PROGRAM p07_memoryCell
VAR
	S0: BOOL;
	S1: BOOL;
	L0: BOOL;
	L1: BOOL;
	L2: BOOL;
	RS_cell: RS;
	SR_cell: SR;
END_VAR

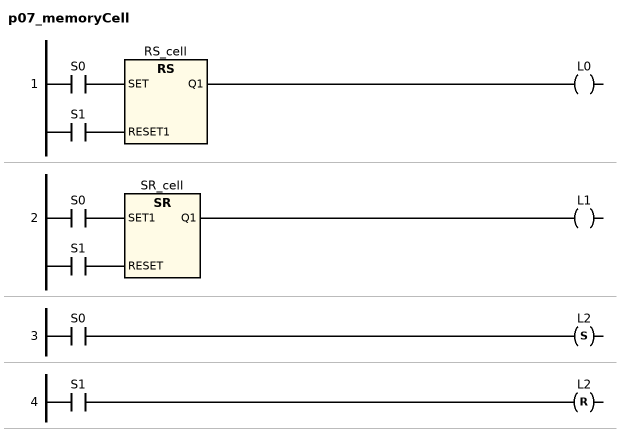
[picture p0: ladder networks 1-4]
// NETWORK 1
RS_cell(SET := S0, RESET1 := S1); // RS
L0 := RS_cell.Q1;

// NETWORK 2
SR_cell(SET1 := S0, RESET := S1); // SR
L1 := SR_cell.Q1;

// NETWORK 3
L2 S= S0;

// NETWORK 4
L2 R= S1;

END_PROGRAM
